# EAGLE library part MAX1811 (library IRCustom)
Maxim MAX1811 USB li-ion battery charger http://www.ladyada.net/library/eagle
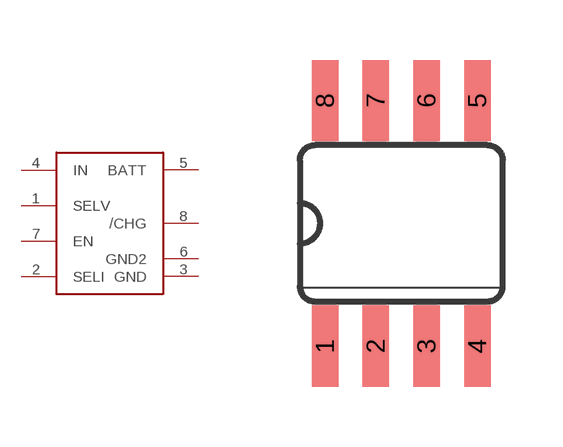
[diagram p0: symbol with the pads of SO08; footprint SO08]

Designator prefix -

## MAX1811SO8  [SO08]
1  SELV
2  SELI
3  GND
4  IN
5  BATT
6  GND2
7  EN
8  /CHG

## Footprint SO08 (pad centres in mm)
smd 0.66 x 2.032: 1 -1.905,-3.073; 2 -0.635,-3.073; 3 0.635,-3.073; 4 1.905,-3.073; 5 1.905,3.073; 6 0.635,3.073; 7 -0.635,3.073; 8 -1.905,3.073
